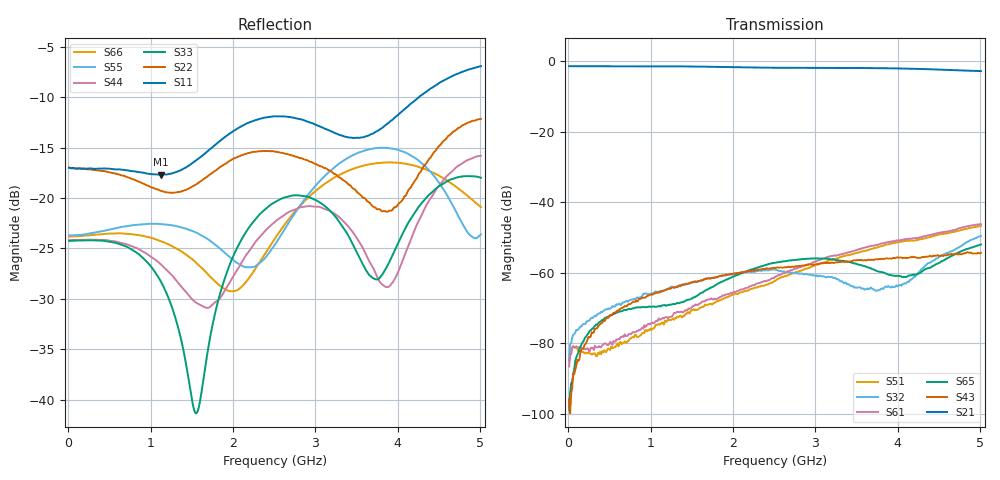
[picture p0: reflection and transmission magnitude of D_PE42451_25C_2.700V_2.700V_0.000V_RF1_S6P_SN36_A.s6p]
! Device ID: PE42451
! Serial: 36
! Insertion: A
! Temp: 25C
! VDD: 2.700
! Control_Hi: 100.000
! Control_Lo: 0.000
! Logic State: RF1
! Port 1: RFC
! Port 2: RF1
! Port 3: RF2
! Port 4: RF3
! Port 5: RF4
! Port 6: RF5
! V1 = 2.70
! V2 = 0.00
! V3 = 0.00
! V4 = 0.00
! IDD: 1.086280e-05
#  Hz  S  RI  R  50
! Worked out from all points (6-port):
!   401 points, 10 MHz to 5.01 GHz, reference 50 ohm
!   strongest paths, dB at 10 MHz, 1.26 GHz, 2.51 GHz, 3.76 GHz, 5.01 GHz:
!     S21: -1.4, -1.5, -1.9, -2.0, -2.8
!     S43: -95.8, -64.2, -58.7, -56.2, -54.4
!     S65: -98.9, -69.0, -57.2, -59.6, -52.0
!     S61: -86.6, -72.4, -61.2, -52.0, -46.2
!     S32: -84.9, -64.0, -59.1, -65.0, -49.6
!     S51: -84.9, -73.2, -62.3, -52.8, -46.7
!   lowest |S11| = -17.7 dB at 1.123 GHz (marker M1), VSWR 1.30, Z = 58.4 - j11.5 ohm
!   |S11| at or under -10 dB: start of sweep to 4.257 GHz
